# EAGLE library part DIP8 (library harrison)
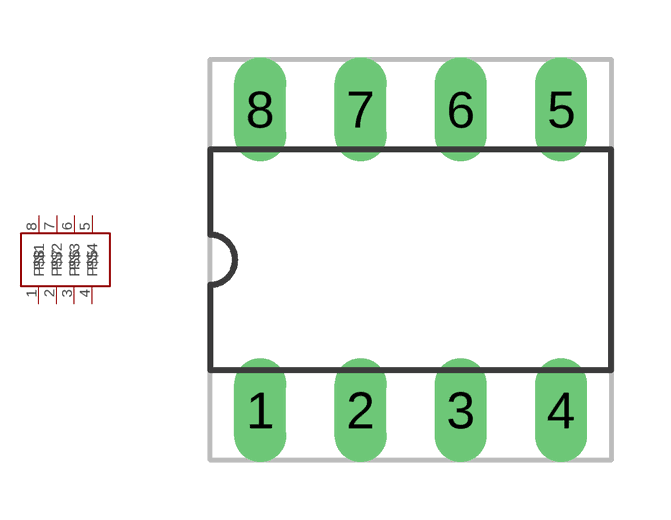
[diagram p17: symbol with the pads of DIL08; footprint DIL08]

Designator prefix -

## DIP8  [DIL08]
1  P$1  pas
2  P$2  pas
3  P$3  pas
4  P$4  pas
5  P$5  pas
6  P$6  pas
7  P$7  pas
8  P$8  pas

## Footprint DIL08 (pad centres in mm)
drill 0.813 long: 1 -3.81,-3.81; 2 -1.27,-3.81; 3 1.27,-3.81; 4 3.81,-3.81; 5 3.81,3.81; 6 1.27,3.81; 7 -1.27,3.81; 8 -3.81,3.81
